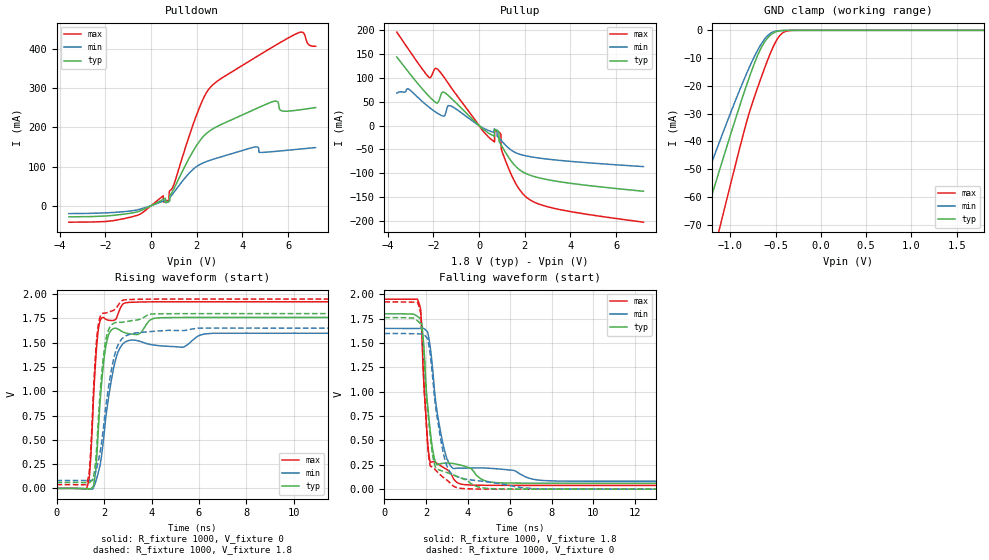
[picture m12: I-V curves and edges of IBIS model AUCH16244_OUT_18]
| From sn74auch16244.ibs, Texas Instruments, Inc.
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[Model]   AUCH16244_OUT_18
Model_type  3-state
Enable   Active-Low
Vref =   0
Rref =   1000
Cref =   30p
Vmeas =   0.9
| variable   typ   min   max
C_comp   5.45pF   4.88pF   5.67pF
| C_pullup   6.31pF   1.00pF   11.78pF
| C_pulldown   6.14pF   1.75pF   14.74pF
| C_tri-state   5.45pF   4.88pF   5.67pF
[Temperature Range]   40   100   -40
| Ambient temperature   25   85   -40
[Voltage range]   1.8   1.65   1.95
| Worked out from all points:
|   slope of the pulldown table from 0 to 0.27 V, typ, clamps not added: 34.2 ohm
|   slope of the pullup table from 0 to 0.27 V, typ, clamps not added: 24.9 ohm
|   GND clamp passes 1 mA (typ) near -0.53 V on its own axis
|   rising waveform, R_fixture 1000, V_fixture 0: 20-80 % time 341ps typ, 554ps min, 261ps max; typ from 0 V to 1.76 V
|   falling waveform, R_fixture 1000, V_fixture 1.8: 20-80 % time 415ps typ, 621ps min, 298ps max; typ from 1.8 V to 0.061 V
|   rising waveform, R_fixture 1000, V_fixture 1.8: 20-80 % time 337ps typ, 558ps min, 256ps max; typ from 0.061 V to 1.8 V
|   falling waveform, R_fixture 1000, V_fixture 0: 20-80 % time 418ps typ, 630ps min, 290ps max; typ from 1.76 V to 0 V
[GND Clamp]
| AUCH16244_OUT_18
|   Voltage   I(typ)   I(min)   I(max)
-3.6V     -322.9mA   -271.3mA   -392.8mA
-1.48V    -89.14mA   -71.99mA   -118.6mA
-1.435V   -84.24mA   -67.93mA   -112.7mA
-1.3V     -69.59mA   -55.85mA   -94.97mA
-1.15V    -53.49mA   -42.68mA   -75.27mA
-1.1V     -48.18mA   -38.36mA   -68.71mA
-830mV    -20.57mA   -16.22mA   -34.06mA
-690mV    -8.335mA   -6.605mA   -19.75mA
-565mV    -1.951mA   -1.255mA   -8.764mA
-490mV    -463.9uA   -245.9uA   -3.576mA
-425mV    -91.38uA   -54.15uA   -985.3uA
1.8V      674.7pA    45.17nA    747.9pA
[Pulldown]
| AUCH16244_OUT_18
|   Voltage   I(typ)   I(min)   I(max)
-3.6V     -28.49mA   -20.22mA   -42.08mA
-1.155V   -21.32mA   -15.05mA   -32.66mA
530mV     16.28mA    11.83mA    25.26mA
780mV     11.06mA    10.81mA    14.1mA
800mV     11.7mA     11.72mA    36.72mA
1.955V    150.3mA    98.42mA    225.9mA
2.625V    193.2mA    116.8mA    304mA
4.56V     246.5mA    149.9mA    378.1mA
5.38V     266.4mA    138.3mA    406.9mA
5.71V     242.1mA    140mA      418.2mA
6.445V    244.1mA    144.1mA    441.1mA
7.2V      250.4mA    148.3mA    406.7mA
[Pullup]
| AUCH16244_OUT_18
|   Voltage   I(typ)   I(min)   I(max)
-3.6V     143.4mA    67.81mA    195.5mA
-2.21V    62.22mA    39.25mA    101.7mA
-1.955V   50.53mA    30.07mA    117.2mA
-1.505V   68.89mA    20.87mA    99.46mA
-1.25V    58.62mA    41.27mA    81.57mA
405mV     -15.38mA   -10.2mA    -23.47mA
835mV     -11.64mA   -24.19mA   -13.09mA
930mV     -37.45mA   -29.05mA   -16.21mA
980mV     -41.44mA   -31.73mA   -49.64mA
1.31V     -67.6mA    -47.58mA   -91.39mA
2.115V    -101.6mA   -63.91mA   -151.5mA
7.2V      -137.4mA   -85.82mA   -202mA
[Ramp]
| AUCH16244_OUT_18
| variable   typ   min   max
dV/dt_r   1.06/3.51E-10   0.96/5.68E-10   1.16/2.71E-10
dV/dt_f   1.04/4.16E-10   0.94/6.33E-10   1.15/3.08E-10
R_load = 1000
[Rising Waveform]
| AUCH16244_OUT_18
R_fixture =   1000
C_fixture =   0
L_fixture =   0
V_fixture =   0
V_fixture_min = 0
V_fixture_max = 0
|   Time   V(typ)   V(min)   V(max)
0s        9.675nV    33.63nV    1.209nV
1.265ns   -5.219mV   -2.631mV   -2.489mV
1.4ns     -6.867mV   -5.066mV   168.6mV
1.545ns   15.95mV    2.388mV    863.3mV
1.775ns   665.7mV    177.7mV    1.657V
2.11ns    1.505V     795.4mV    1.738V
2.495ns   1.649V     1.331V     1.741V
2.905ns   1.601V     1.51V      1.912V
4.505ns   1.758V     1.466V     1.922V
34.99ns   1.761V     1.597V     1.922V
[Falling Waveform]
| AUCH16244_OUT_18
R_fixture =   1000
C_fixture =   0
L_fixture =   0
V_fixture =   1.8
V_fixture_min = 1.65
V_fixture_max = 1.95
|   Time   V(typ)   V(min)   V(max)
0s        1.8V       1.65V      1.95V
1.605ns   1.77V      1.649V     1.938V
1.8ns     1.669V     1.652V     1.542V
2.025ns   960mV      1.623V     614.5mV
2.18ns    621.4mV    1.476V     284.4mV
2.465ns   267.4mV    877.6mV    271.2mV
2.865ns   266.8mV    406.7mV    216.8mV
3.655ns   246.5mV    215.4mV    52.01mV
5.625ns   64.44mV    204.6mV    38.92mV
34.99ns   61.09mV    81.02mV    38.7mV
[Rising Waveform]
| AUCH16244_OUT_18
R_fixture =   1000
C_fixture =   0
L_fixture =   0
V_fixture =   1.8
V_fixture_min = 1.65
V_fixture_max = 1.95
|   Time   V(typ)   V(min)   V(max)
0s        61.05mV    81.01mV    38.68mV
1.26ns    59.3mV     81.33mV    38.19mV
1.395ns   60.15mV    81.75mV    224mV
1.545ns   99.24mV    94.43mV    942.6mV
1.755ns   692.1mV    276.2mV    1.678V
1.92ns    1.226V     513.8mV    1.8V
2.085ns   1.54V      864.1mV    1.807V
2.45ns    1.705V     1.376V     1.842V
2.84ns    1.714V     1.559V     1.941V
34.99ns   1.8V       1.65V      1.95V
[Falling Waveform]
| AUCH16244_OUT_18
R_fixture =   1000
C_fixture =   0
L_fixture =   0
V_fixture =   0
V_fixture_min = 0
V_fixture_max = 0
|   Time   V(typ)   V(min)   V(max)
0s        1.761V     1.597V     1.922V
1.595ns   1.727V     1.594V     1.911V
1.79ns    1.638V     1.593V     1.608V
1.93ns    1.254V     1.578V     925.5mV
2.17ns    591.8mV    1.412V     259.3mV
2.43ns    232.5mV    879.2mV    199.8mV
2.82ns    183mV      369.2mV    120.4mV
3.475ns   131.2mV    129.3mV    15.24mV
5.52ns    2.61mV     56.38mV    293.7uV
34.99ns   36.49uV    4.007uV    15.84uV
